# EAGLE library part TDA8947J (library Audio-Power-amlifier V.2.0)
The TDA8947J contains four identical audio power amplifiers. The TDA8947J can be used as: four Single-Ended (SE: 1 W to 25 W; BTL: 4 W to 50 W)) channels with a fixed gain of 26 dB, two times Bridge-Tied Load (BTL) channels with a fixed gain of 32 dB or two times SE channels (26 dB gain) plus one BTL channel (32 dB gain) operating as a 2.1 system.
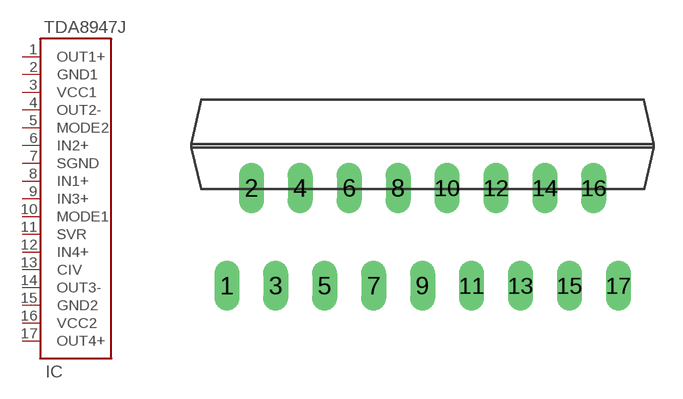
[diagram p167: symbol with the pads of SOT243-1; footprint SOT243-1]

Designator prefix IC

## TDA8947J  [SOT243-1]
1  OUT1+  out
2  GND1  pwr
3  VCC1  pwr
4  OUT2-  out
5  MODE2  in
6  IN2+  in
7  SGND  pwr
8  IN1+  in
9  IN3+  in
10  MODE1  in
11  SVR
12  IN4+  in
13  CIV  in
14  OUT3-  out
15  GND2  out
16  VCC2  pwr
17  OUT4+  out

## Footprint SOT243-1 (pad centres in mm)
DBS17P: plastic DIL-bent-SIL power package; 17 leads (lead length 7.7 mm)
drill 0.8 long: 1 -10.16,-5.08; 2 -8.89,0; 3 -7.62,-5.08; 4 -6.35,0; 5 -5.08,-5.08; 6 -3.81,0; 7 -2.54,-5.08; 8 -1.27,0; 9 0,-5.08; 10 1.27,0; 11 2.54,-5.08; 12 3.81,0; 13 5.08,-5.08; 14 6.35,0; 15 7.62,-5.08; 16 8.89,0; 17 10.17,-5.08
